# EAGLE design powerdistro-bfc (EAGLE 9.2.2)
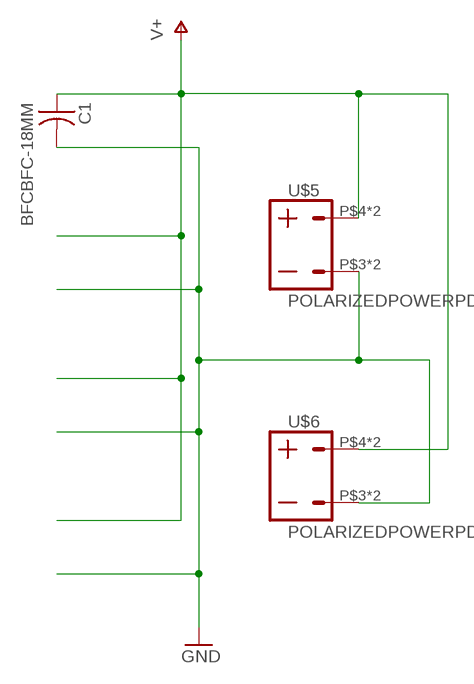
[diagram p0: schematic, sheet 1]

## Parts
C1  BFCBFC-18MM  [BFC-18MM-7-5MM]
U$5  POLARIZEDPOWERPDB  [PDBCONN]
U$6  POLARIZEDPOWERPDB  [PDBCONN]

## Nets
GND: C1.P$1 U$5.P$3 U$5.P$6 U$6.P$3 U$6.P$6
V+: C1.P$2 U$5.P$4 U$5.P$5 U$6.P$4 U$6.P$5

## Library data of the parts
C1 = power:BFC
U$5 U$6 = connector:POLARIZEDPOWER

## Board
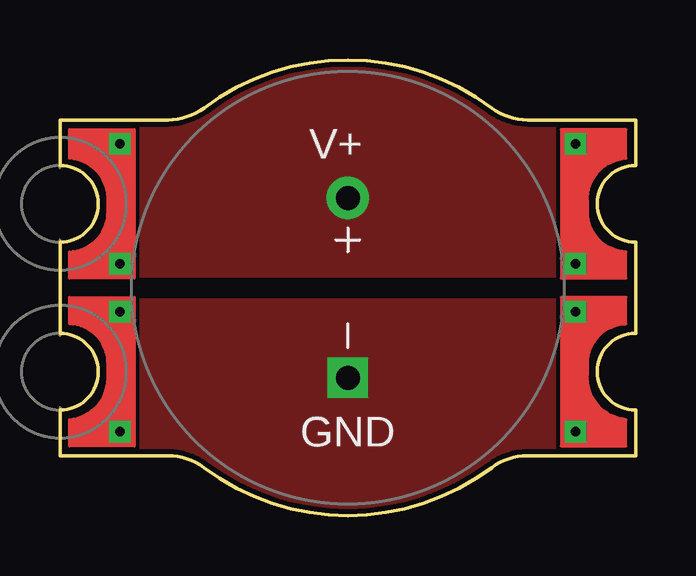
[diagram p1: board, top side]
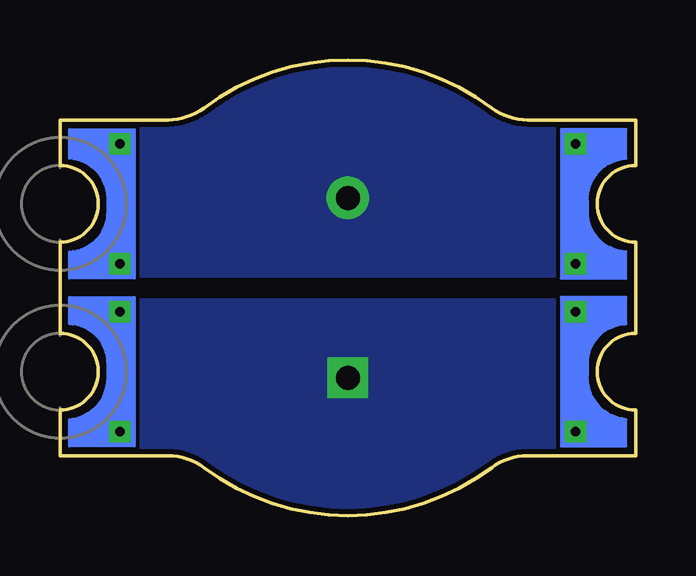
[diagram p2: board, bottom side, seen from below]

Size 24 x 19 mm. Coordinates in mm from the lower left corner, seen from the top.
Outline: 0,7.6 0,11.4 arc90 1.6,13 arc90 0,14.6 0,16.5 4.5,16.5 arc37 6,17 arc-37 12,19 arc-37 18,17 arc37 19.5,16.5 24,16.5 24,14.6 arc90 22.4,13 arc90 24,11.4 24,7.6 arc90 22.4,6 arc90 24,4.4 24,2.5 19.5,2.5 arc37 18,2 arc-37 12,0 arc-37 6,2 arc37 4.5,2.5 0,2.5 0,4.4 arc90 1.6,6 arc90 0,7.6
Copper layers (1*16): Top 0.035mm / dielectric 1.5mm / Bottom 0.035mm
Design rules "default *": minimum track width 6mil, minimum drill 0.35mm, track to track 6mil, track to pad 6mil, pad to pad 6mil, via to via 6mil, smd to smd 6mil, copper to edge 8mil, drill to drill 6mil, minimum pad ring 10mil, minimum via ring 8mil, stop-mask expansion 4mil, vias tented up to drill 0mil, thermal gap 10mil

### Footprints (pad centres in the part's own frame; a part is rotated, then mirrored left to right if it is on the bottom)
BFC-18MM-7-5MM = drill 1 pad 1.676 square: P$1 -3.75,0 | drill 1 pad 1.778: P$2 3.75,0
PDBCONN = drill 0.4 square: P$3 2.5,2.5; P$4 2.5,4.5; P$5 2.5,9.5; P$6 2.5,-2.5

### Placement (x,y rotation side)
C1  12,9.5 90 top
U$5  0,6 0 top
U$6  24,6 0 bottom

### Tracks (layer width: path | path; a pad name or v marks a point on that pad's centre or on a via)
GND
  pour Top: -1,9 26.5,9 26.5,-1 -1,-1
  pour Bottom: -1.5,9 27,9 27,-1.5 -1.5,-1.5
V+
  pour Top: -1,10 26.5,10 26.5,20.5 -1,20.5
  pour Bottom: -1.5,10 27,10 27,21 -1.5,21

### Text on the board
tPlace: V+ | GND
